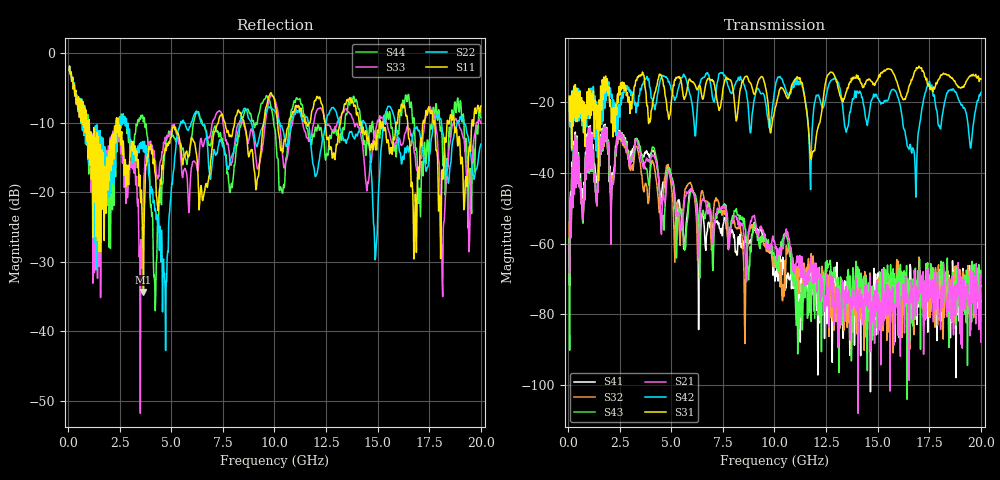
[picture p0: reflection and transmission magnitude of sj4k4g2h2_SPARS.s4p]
! FILE: E:\users\goganessyan\GBX_Backplane\FR408_backplane\1m_OUTBOUND_FEXT\sj4k4g2h2_SPARS.s4p
# MHZ S RI R 50.00
! FREQ  S11  S12  S13  S14
!  S21  S22  S23  S24
!  S31  S32  S33  S34
!  S41  S42  S43  S44
!  REAL  IMAG  REAL  IMAG  REAL  IMAG  REAL  IMAG
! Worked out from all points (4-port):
!   799 points, 50 MHz to 20 GHz, reference 50 ohm
!   strongest paths, dB at 50 MHz, 5.025 GHz, 10.03 GHz, 15.03 GHz, 20 GHz:
!     S31: -18.3, -18.7, -21.7, -13.3, -13.5
!     S42: -19.1, -16.6, -16.1, -18.9, -17.2
!     S21: -60.1, -42.0, -60.3, -74.4, -87.9
!     S43: -58.7, -41.3, -63.5, -76.3, -67.7
!     S32: -53.9, -44.6, -65.0, -71.0, -76.7
!     S41: -61.6, -41.7, -70.6, -68.2, -71.8
!   lowest |S11| = -34.3 dB at 3.65 GHz (marker M1), VSWR 1.04, Z = 51.3 + j1.48 ohm
!   |S11| at or under -10 dB: 1.027 GHz to 2.329 GHz (1.302 GHz wide, 77.6 % of centre); 2.437 GHz to 7.278 GHz (4.841 GHz wide, 99.7 % of centre); 8.529 GHz to 9.481 GHz (952.2 MHz wide, 10.6 % of centre)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
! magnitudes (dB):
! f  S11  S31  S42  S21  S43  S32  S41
! 50 MHz  -2.5  -18.3  -19.1  -60.1  -58.7  -53.9  -61.6
! 1 GHz  -12.9  -16.2  -16.5  -27.3  -28.3  -28.9  -26.9
! 3.65 GHz  -34.3  -12.2  -14.4  -38.6  -36.9  -45.1  -35.4
! 4.225 GHz  -17.3  -17.1  -21.2  -36.1  -34.2  -39.8  -35.3
! 11.2 GHz  -8.0  -13.5  -14.1  -66.7  -84.0  -65.4  -81.6
! 16.82 GHz  -20.3  -11.1  -40.5  -70.7  -66.9  -74.3  -72.9
! 20 GHz  -7.6  -13.5  -17.2  -87.9  -67.7  -76.7  -71.8
